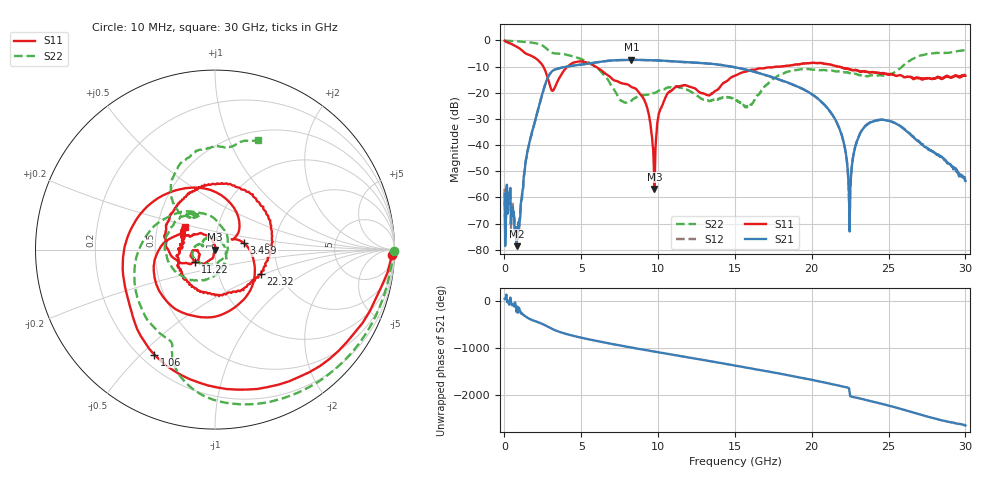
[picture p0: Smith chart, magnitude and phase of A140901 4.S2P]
!  2-Port S-parameters saved by WinCal
! VAR MeasName=S-Parameters (CALIBRATED_DATA) read from VNA (N5244A)
! VAR MeasDate=11/3/2014 9:26:49 AM
! VAR NAME=A140901 4
! VAR FILENAME=A140901 4.S2P
! VAR DATE=11/3/2014 9:26:49 AM
! VAR PHYS_PORTS=1,2
# Hz S RI R 50
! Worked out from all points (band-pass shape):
!   801 points, 10 MHz to 30 GHz, reference 50 ohm
!   highest |S21| = -7.40 dB at 8.257 GHz (marker M1); lowest = -78.6 dB at 797.2 MHz (marker M2)
!   |S21| within 3 dB of the highest: 3.721 GHz to 15.11 GHz (11.39 GHz wide, 121 % of centre)
!   lowest |S11| = -56.8 dB at 9.757 GHz (marker M3), VSWR 1.00, Z = 50.1 - j0.0545 ohm
!   |S11| at or under -10 dB: 2.528 GHz to 4.107 GHz (1.579 GHz wide, 47.6 % of centre); 5.934 GHz to 17.76 GHz (11.83 GHz wide, 99.8 % of centre); 21.75 GHz to end of sweep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
!   |S22| runs from -25.6 to 0.0 dB; largest |S21 - S12| = 0.0037
!   S11 on the Smith chart (normalised r, x): 10 MHz: 24, -54; 1.06 GHz: 0.25, -0.55; 3.459 GHz: 1.38, +0.10; 11.22 GHz: 0.79, -0.11; 22.32 GHz: 1.60, -0.48; 30 GHz: 0.69, +0.18
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1e7  0.9861 -0.0305  0.000834 0.00082  0.0014 -0.000431  0.9982 -0.00866
7.972375e8  -0.0409 -0.7565  -5.8e-05 0.000102  -6.03e-05 0.000262  0.8377 -0.4729
1.05965e9  -0.3395 -0.5848  -0.000104 0.000732  -0.000196 0.000687  0.7395 -0.5982
1.8094e9  -0.4942 0.0475  0.012 -0.0141  0.012 -0.0141  0.3404 -0.8393
3.45885e9  0.1626 0.0351  0.0801 0.2776  0.0795 0.2773  -0.2859 -0.4821
5.033325e9  -0.2603 -0.2975  0.1318 -0.3206  0.1315 -0.321  -0.4354 -0.0341
6.720262e9  -0.1995 0.0848  -0.4064 0.00189  -0.4057 0.00152  -0.0122 0.1802
8.25725e9  -0.0967 0.0862  0.0393 0.4247  0.0394 0.4231  0.0216 -0.0661
9.231925e9  -0.0171 0.0551  0.3723 0.1961  0.372 0.1962  -0.0451 -0.08
9.75675e9  0.00135 -0.000544  0.4156 -0.0163  0.415 -0.0156  -0.0623 -0.0768
1.001916e10  -0.00869 -0.034  0.3961 -0.1224  0.3955 -0.122  -0.0761 -0.0779
1.121876e10  -0.1118 -0.0689  0.0377 -0.3928  0.0381 -0.3928  -0.1273 -0.0278
1.298068e10  -0.0955 -0.0109  -0.3668 0.016  -0.3672 0.0158  -0.0692 0.0266
1.5005e10  -0.2002 -0.0678  0.152 0.2659  0.154 0.2643  -0.0274 0.0688
1.721676e10  -0.2694 0.1406  0.0712 -0.196  0.0697 -0.1953  -0.0239 -0.1548
2.002832e10  0.0632 0.3693  -0.0375 0.0846  -0.0379 0.0845  -0.259 0.0921
2.167778e10  0.3152 0.0324  0.0253 -0.000948  0.0249 -0.000787  -0.1662 0.194
2.231506e10  0.2571 -0.1361  0.0027 -0.00304  0.00269 -0.00307  -0.133 0.2051
2.253999e10  0.2223 -0.1726  -0.00109 0.00185  -0.00114 0.00194  -0.1221 0.1983
2.336471e10  0.0401 -0.2548  0.0109 0.018  0.0109 0.0181  -0.1009 0.1946
2.501416e10  -0.1922 -0.1089  0.00773 -0.0279  0.00782 -0.028  -0.1298 0.1832
3e10  -0.1685 0.1266  -0.00154 -0.00137  -0.00134 -0.00151  0.2416 0.6121
